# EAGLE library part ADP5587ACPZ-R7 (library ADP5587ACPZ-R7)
Analog Devices ADP5587ACPZ-R7, 18-channel 18bit I/O Expander 400kHz, I2C, 24-Pin LFCSP WQ Source: Datasheet
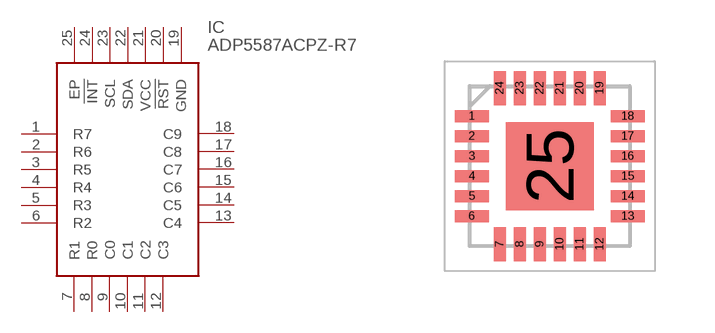
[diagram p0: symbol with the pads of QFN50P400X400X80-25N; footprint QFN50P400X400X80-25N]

Designator prefix IC

## ADP5587ACPZ-R7 (Description: Analog Devices ADP5587ACPZ-R7, 18-channel 18bit I/O Expander 400kHz, I2C, 24-Pin LFCSP WQ; Height: 0.8mm; Manufacturer_Name: Analog Devices; Manufacturer_Part_Number: ADP5587ACPZ-R7; Mouser_Part_Number: 584-ADP5587ACPZ-R7; Mouser_Price-Stock: https://www.mouser.com/Search/Refine.aspx?Keyword=584-ADP5587ACPZ-R7)  [QFN50P400X400X80-25N]
1  R7
2  R6
3  R5
4  R4
5  R3
6  R2
7  R1
8  R0
9  C0
10  C1
11  C2
12  C3
13  C4
14  C5
15  C6
16  C7
17  C8
18  C9
19  GND
20  !RST
21  VCC
22  SDA
23  SCL
24  !INT
25  EP

## Footprint QFN50P400X400X80-25N (pad centres in mm)
LFCSP_WQ-1
smd 0.85 x 0.3: 1 -1.95,1.25; 2 -1.95,0.75; 3 -1.95,0.25; 4 -1.95,-0.25; 5 -1.95,-0.75; 6 -1.95,-1.25; 13 1.95,-1.25; 14 1.95,-0.75; 15 1.95,-0.25; 16 1.95,0.25; 17 1.95,0.75; 18 1.95,1.25
smd 0.3 x 0.85: 7 -1.25,-1.95; 8 -0.75,-1.95; 9 -0.25,-1.95; 10 0.25,-1.95; 11 0.75,-1.95; 12 1.25,-1.95; 19 1.25,1.95; 20 0.75,1.95; 21 0.25,1.95; 22 -0.25,1.95; 23 -0.75,1.95; 24 -1.25,1.95
smd 2.2 x 2.2: 25 0,0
